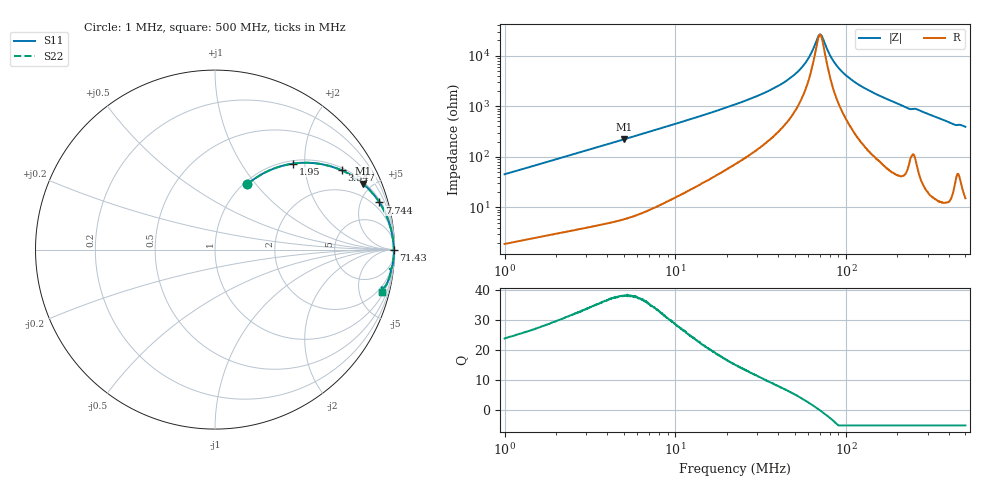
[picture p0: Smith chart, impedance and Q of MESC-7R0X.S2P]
!s-Parameter Generated by FASTRON Sdn. Bhd.
!FASTRON P/N : MESC-7R0X
!Keysight Technologies,E4991B,MY54100416,A.01.15
!Date: Mon Mar 16 10:43:48 2026
!Version  : Rev00 Mon Mar 16 10:43:48 2026
!Data & Calibration Information:
!PortZ  Port1:50+j0  Port2:50+j0
!When reading, reference impedance value at option line is always used.
!Remarks : This data is being provided solely for informational purposes.
!Freq	S11	S21	S12	S22
# Hz S dB R 50
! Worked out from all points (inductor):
!   1601 points, 1 MHz to 500 MHz, reference 50 ohm
!   read as one part in series: L = 7.15 uH near 1.032 MHz
!   highest Q = 38.1 at 4.993 MHz (marker M1), where L = 7.05 uH
!   self-resonance near 70.32 MHz
!   S11 on the Smith chart (normalised r, x): 1 MHz: 1.04, +0.90; 1.95 MHz: 1.06, +1.74; 3.547 MHz: 1.09, +3.14; 7.744 MHz: 1.21, +6.90; 71.43 MHz: open; 500 MHz: 1.30, -7.85
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1000000  -7.83 63.7  -0.94 -23.9  -0.94 -23.9  -7.83 63.7
1950470  -3.80 47.9  -2.59 -40.2  -2.59 -40.2  -3.80 47.9
2820919  -2.27 37.9  -4.22 -50.3  -4.22 -50.3  -2.27 37.9
3547441  -1.59 32.0  -5.51 -56.4  -5.51 -56.4  -1.59 32.0
4992965  -0.89 24.1  -7.79 -64.4  -7.79 -64.4  -0.89 24.1
7744141  -0.42 16.0  -11.18 -72.3  -11.18 -72.3  -0.42 16.0
7957584  -0.40 15.6  -11.41 -72.7  -11.41 -72.7  -0.40 15.6
2.236068e7  -0.09 5.2  -20.77 -81.0  -20.77 -81.0  -0.09 5.2
3.388275e7  -0.06 3.0  -25.61 -81.3  -25.61 -81.3  -0.06 3.0
4.499032e7  -0.04 1.7  -30.22 -79.7  -30.22 -79.7  -0.04 1.7
5.484648e7  -0.04 1.0  -35.26 -75.0  -35.26 -75.0  -0.04 1.0
5.927696e7  -0.04 0.7  -38.30 -69.9  -38.30 -69.9  -0.04 0.7
6.307767e7  -0.03 0.4  -41.53 -61.3  -41.53 -61.3  -0.03 0.4
6.843836e7  -0.03 0.1  -47.36 -26.0  -47.36 -26.0  -0.03 0.1
7.142578e7  -0.03 -0.1  -48.22 13.9  -48.22 13.9  -0.03 -0.1
8.278574e7  -0.03 -0.6  -38.78 71.5  -38.78 71.5  -0.03 -0.6
9.707707e7  -0.03 -1.3  -33.01 80.0  -33.01 80.0  -0.03 -1.3
1.239906e8  -0.03 -2.3  -27.78 83.3  -27.78 83.3  -0.03 -2.3
1.77937e8  -0.05 -4.3  -22.59 83.4  -22.59 83.4  -0.05 -4.3
2.299316e8  -0.11 -6.2  -19.33 80.2  -19.33 80.2  -0.11 -6.2
4.247389e8  -0.30 -12.6  -13.22 74.8  -13.22 74.8  -0.30 -12.6
5e8  -0.35 -14.1  -12.24 73.6  -12.24 73.6  -0.35 -14.1
